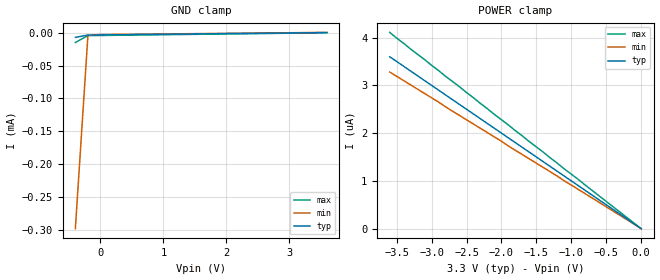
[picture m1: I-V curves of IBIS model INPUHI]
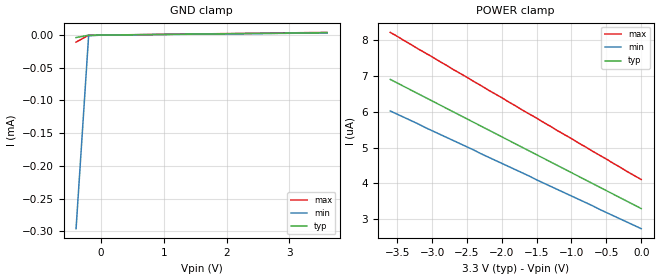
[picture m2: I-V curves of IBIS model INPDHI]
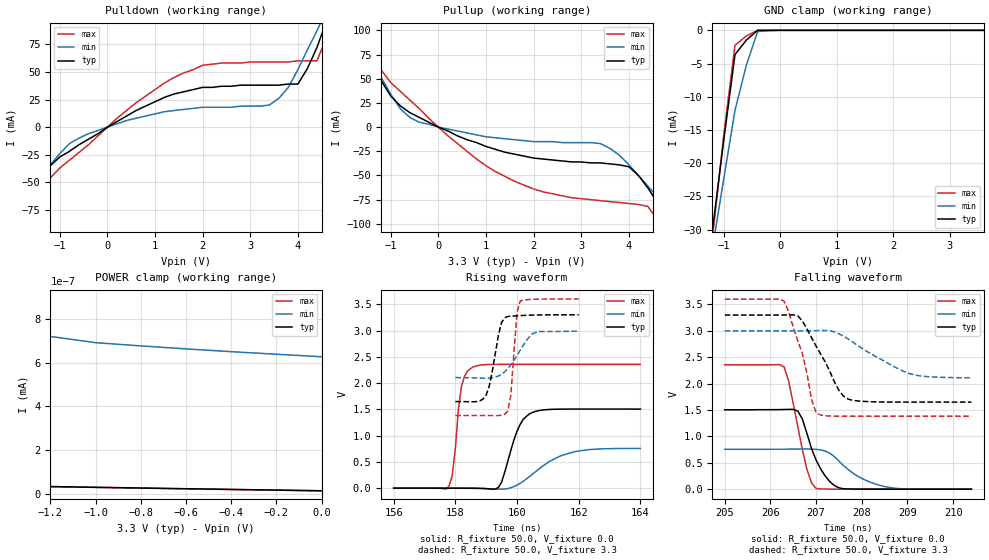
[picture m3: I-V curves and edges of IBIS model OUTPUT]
|   Texas Instruments Incorporated
|   Data Transmissions Products
|   IBIS Model for ISO723x4x
|   16DW SOIC Package
[IBIS Ver]   3.2
[Comment char]   |_char
[File name]   iso7240cf_3.ibs
[File Rev]   1.0
[Date]   10July08
[Source]   File originated at Texas Instruments Incorporated.
   Data Transmission Products Group.
[Notes]
[Disclaimer]
(C) Copyright Texas Instruments Incorporated 2002
   All rights reserved
  Texas Instruments Incorporated hereby grants the user of this IBIS
model a non-exclusive, nontransferable license to use this IBIS model
under the following terms.  Before using this IBIS model, the user
should read this license.  If the user does not accept these terms,
the IBIS model should be returned to Texas Instruments within 30 days.
  The user is granted this license only to use the IBIS model and
is not granted rights to sell, load, rent, lease or license the IBIS
model in whole or in part, or in modified form to anyone other than
user.  User may modify the IBIS model to suit its specific applications
but rights to derivative works and such modifications shall belong to
Texas Instruments.
  This IBIS model is provided on an "AS IS" basis and Texas Instruments
makes absolutely no warranty with respect to the information contained
herein.  TEXAS INSTRUMENTS DISCLAIMS AND CUSTOMER WAIVES ALL WARRANTIES,
EXPRESS OR IMPLIED, INCLUDING WARRANTIES OF MERCHANTABILITY OR FITNESS
FOR A PARTICULAR PURPOSE. The entire risk as to quality and performance
is with the Customer. ACCORDINGLY, IN NO EVENT SHALL THE COMPANY BE LIABLE
FOR ANY DAMAGES, WHETHER IN CONTRACT OR TORT,INCLUDING ANY LOST PROFITS
OR OTHER INCIDENTAL, CONSEQUENTIAL, EXEMPLARY, OR PUNITIVE DAMAGES ARISING
OUT OF THE USE OR APPLICATION OF THE IBIS model provided in this package.
Further, Texas Instruments reserves the right to discontinue or make changes
without notice to any product herein to improve reliability, function, or
design. Texas Instruments does not convey any license under patent rights
or any other intellectual property rights, including those of third parties.
Contact Texas Instruments at ATTN:DATA TRANSMISSIONS
[Copyright]   Copyright 2002, Texas Instruments, All Rights Reserved
[Component]   ISO7240DW
[Manufacturer]  Texas Instruments Incorporated
[Package]
|   typ   min   max
R_pkg   0.04817   0.03432   0.09530
L_pkg   2.4595nH   1.6904nH   4.7034nH
C_pkg   0.847pF   0.428pF   1.397pF
[Pin]   signal_name   model_name   R_pin   L_pin   C_pin
1   VCC1   POWER   0.03455  3.39778n  0.89677p
2   GND1   GND   0.03432  3.12613n  0.84706p
3   INA   INPUHI   0.04265  1.85523n  0.57831p
4   INB   INPUHI   0.03948  1.69049n  0.59300p
5   INC   INPUHI   0.03943  1.70546n  0.55709p
6   IND   INPUHI   0.04257  1.86953n  0.56379p
7   DISABLE   INPDHI   0.04783  1.99000n  0.60148p
8   GND1   GND   0.03740  4.70338n  1.39696p
9   GND2   GND   0.03763  4.61305n  1.39587p
10   CTRL   INPUHI   0.04703  2.01514n  0.58483p
11   OUTD   OUTPUT   0.07132  2.45946n  0.43321p
12   OUTC   OUTPUT   0.06147  2.13194n  0.42769p
13   OUTB   OUTPUT   0.07288  2.39260n  0.48001p
14   OUTA   OUTPUT   0.09530  3.03704n  0.47622p
15   GND2   GND   0.04817  4.23145n  0.93567p
16   VCC2   POWER   0.04790  4.51154n  0.99405p
| Models and submodels in the file (3): INPUHI (Input), INPDHI (Input), OUTPUT (3-state)
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|   Driver Enable
[Model]   INPUHI
Model_type   Input
|Signals   INA,INB,INC,IND,CTRL
Vinh = 2.0
Vinl = 0.8
|   typ   min   max
C_comp   1.3pF   1.1pF   1.5pF
|   typ   min   max
[Temperature Range]   27   -40   125
[Voltage range]   3.3V   3.0V   3.6V
[GND_clamp]
|   Voltage   I(typ)   I(min)   I(max)
-400mV    -7.04uA    -298uA     -14.8uA
-200mV    -3.5uA     -3.91uA    -4.34uA
0V        -3.3uA     -2.74uA    -4.11uA
3.6V      300nA      549nA      14.4pA
[Power_clamp]
| Note that the[POWER_clamp]voltage table is referenced to Vcc
| and is calculated using Vtable=Vcc - Vmeasured.
|   Voltage   I(typ)   I(min)   I(max)
-3.6V     3.6uA      3.28uA     4.11uA
-2.9V     2.9uA      2.65uA     3.31uA
-2.8V     2.8uA      2.55uA     3.19uA
0V        0A         0A         0A
|   Driver Input / Receiver Enable Model
[Model]   INPDHI
Model_type   Input
|Signals   DISABLE
Vinh = 2.0
Vinl = 0.8
|   typ   min   max
C_comp   1.3pF   1.1pF   1.5pF
|   typ   min   max
[Temperature Range]   27   -40   125
[Voltage range]   3.3V   3.0V   3.6V
[GND_clamp]
|   Voltage   I(typ)   I(min)   I(max)
-400mV    -3.79uA    -296uA     -10.8uA
-200mV    -202nA     -1.2uA     -230nA
0V        0A         0A         0A
3.6V      3.6uA      3.28uA     4.11uA
[Power_clamp]
| Note that the[POWER_clamp]voltage table is referenced to Vcc
| and is calculated using Vtable=Vcc - Vmeasured.
|   Voltage   I(typ)   I(min)   I(max)
-3.6V     6.9uA      6.02uA     8.21uA
-500mV    3.8uA      3.19uA     4.68uA
-200mV    3.5uA      2.92uA     4.33uA
0V        3.3uA      2.74uA     4.11uA
[Model]   OUTPUT
Model_type   3-state
| Signals   OUT
Vmeas = 2.2V   |Reference voltage for timing measurements
Cref = 15pF   |Timing specification test load capacitance value
Vref = 0   |Timing specification test load voltage; GND
| variable   typ   min   max
C_comp   2.1pF   1.7pF   2.5pF
|   typ   min   max
[Temperature Range]   25.0   -40   125
[Voltage range]   3.3V   3.0V   3.6V
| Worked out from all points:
|   slope of the pulldown table from 0 to 0.495 V, typ, clamps not added: 40 ohm
|   slope of the pullup table from 0 to 0.495 V, typ, clamps not added: 45.4 ohm
|   GND clamp passes 1 mA (typ) near -0.54 V on its own axis
|   POWER clamp passes 1 mA (typ) near -2.27 V on its own axis
|   rising waveform, R_fixture 50.0, V_fixture 0.0: 20-80 % time 494ps typ, 1.13ns min, 242ps max; typ from 0 V to 1.5 V
|   falling waveform, R_fixture 50.0, V_fixture 0.0: 20-80 % time 416ps typ, 716ps min, 336ps max; typ from 1.5 V to 0 V
|   rising waveform, R_fixture 50.0, V_fixture 3.3: 20-80 % time 308ps typ, 597ps min, 168ps max; typ from 1.65 V to 3.3 V
|   falling waveform, R_fixture 50.0, V_fixture 3.3: 20-80 % time 592ps typ, 1.04ns min, 405ps max; typ from 3.3 V to 1.65 V
[Pulldown]
|   Voltage  I(typ)   I(min)   I(max)
-3.6V     -213mA     -167mA     -286mA
-2.2V     -106mA     -89mA      -137mA
-1.8V     -76mA      -66mA      -95mA
-1.2V     -35mA      -34mA      -46mA
-600mV    -16mA      -10mA      -23mA
2V        36mA       18mA       56mA
3.4V      38mA       20mA       59mA
4V        39mA       52mA       60mA
4.4V      72mA       87mA       60mA
4.6V      96mA       106mA      81mA
4.8V      120mA      124mA      106mA
7.5V      465mA      379mA      575mA
[Pullup]
|   Voltage   I(typ)  I(min)  I(max)
| Note that the[Pullup]voltage table is referenced to Vcc
| and is calculated using Vtable=Vcc - Vmeasured.
-3.6V     345mA      272mA      457mA
-2V       144mA      123mA      182mA
-1.5V     83mA       78mA       100mA
-1.2V     48mA       51mA       59mA
-600mV    15mA       10mA       28mA
800mV     -16mA      -8mA       -33mA
2V        -32mA      -15mA      -64mA
3.4V      -37mA      -17mA      -76mA
4V        -41mA      -39mA      -79mA
4.4V      -63mA      -61mA      -82mA
5V        -108mA     -95mA      -134mA
7.2V      -281mA     -221mA     -373mA
[GND_clamp]
|   Voltage   I(typ)   I(min)   I(max)
| Outputs in High Impedance (off)
-3.6V     -213mA     -167.2mA   -285.4mA
-1.2V     -30.16mA   -32.94mA   -31.43mA
-1.1V     -23.41mA   -27.68mA   -23.65mA
-1V       -16.66mA   -22.42mA   -15.87mA
-800mV    -3.66mA    -12.05mA   -2.249mA
-600mV    -1.479mA   -5.279mA   -861.1uA
-400mV    -1.657uA   -187.7uA   -4.797uA
0V        -40.79pA   -10.95nA   -39.6pA
3.6V      17.57pA    663pA      12.68pA
[POWER_clamp]
|   Voltage  I(typ)   I(min)   I(max)
| Note that the [POWER_clamp] voltage table is referenced to Vcc
| and is calculated using Vtable = Vcc - Vmeasured.
| Outputs in Tri-state.
-3.6V     130.9mA    132.2mA    129.3mA
-2.2V     594.7uA    10.13mA    942.3pA
-2.1V     8.158nA    6.126mA    495.1pA
-2V       5.434nA    2.119mA    47.98pA
-1.8V     1.376nA    388.9uA    43.35pA
-1.7V     41.24pA    194.6uA    41.32pA
-1.5V     37.53pA    132.3nA    37.35pA
-1.4V     35.76pA    755.1pA    35.42pA
-1.2V     32.25pA    720.1pA    31.79pA
-1V       28.85pA    691.4pA    28.37pA
-400mV    19.15pA    650.1pA    18.72pA
0V        12.94pA    627pA      12.68pA
[Ramp]
|   typ   min   max
dV/dt_r   0.903V/0.494ns   0.454V/1.13ns   1.414V/0.242ns
dV/dt_f   0.903V/0.416ns   0.453V/0.717ns  1.414V/0.336ns
R_load = 50
[Rising Waveform]
R_fixture = 50.0
V_fixture = 0.0
C_fixture = 0p
L_fixture = 0n
|   V(typ)   V(min)   V(max)
156ns     489.7pV    12.09nV    431.9pV
157.8ns   17.01uV    282.3uV    42.76mV
157.9ns   27.86uV    217.4uV    238.3mV
158.2ns   89.93uV    -788.4uV   1.94V
158.6ns   -99.63uV   -4.419mV   2.312V
159.4ns   15.91mV    -17.3mV    2.357V
160ns     1.083V     58.82mV    2.357V
160.5ns   1.441V     266mV      2.357V
161.9ns   1.506V     698.7mV    2.357V
164ns     1.505V     756mV      2.357V
[Falling Waveform]
R_fixture = 50.0
V_fixture = 0.0
C_fixture = 0p
L_fixture = 0n
|   V(typ)   V(min)   V(max)
205ns     1.505V     755.2mV    2.357V
206.3ns   1.51V      757.4mV    2.318V
206.4ns   1.512V     758.3mV    2.047V
206.6ns   1.481V     760.6mV    1.187V
206.8ns   1.057V     762mV      375.6mV
207ns     553.1mV    755.1mV    12.03mV
207.3ns   143.1mV    683mV      796.9uV
207.6ns   7.515mV    447.7mV    36.71uV
208.5ns   197.3uV    48.97mV    -2.819uV
210.4ns   -4.04uV    324.3uV    303.2nV
[Rising Waveform]
R_fixture = 50.0
V_fixture = 3.3
V_fixture_min = 3.0
V_fixture_max = 3.6
C_fixture = 0p
L_fixture = 0n
|   V(typ)   V(min)  V(max)
158ns     1.649V     2.106V     1.383V
159ns     1.774V     2.093V     1.382V
159.1ns   1.943V     2.094V     1.382V
159.5ns   3.156V     2.171V     1.389V
159.7ns   3.268V     2.277V     1.468V
159.8ns   3.274V     2.348V     1.768V
160ns     3.282V     2.527V     3.341V
160.1ns   3.285V     2.625V     3.559V
160.6ns   3.296V     2.964V     3.597V
162ns     3.3V       2.989V     3.6V
[Falling Waveform]
R_fixture = 50.0
V_fixture = 3.3
V_fixture_min = 3.0
V_fixture_max = 3.6
C_fixture = 0p
L_fixture = 0n
|   V(typ)   V(min)  V(max)
205ns     3.3V       3V         3.6V
206.3ns   3.3V       3V         3.563V
206.6ns   3.286V     3V         2.812V
206.7ns   3.187V     3V         2.569V
206.9ns   2.874V     3.002V     1.705V
207.1ns   2.561V     3.006V     1.404V
207.5ns   1.872V     2.947V     1.383V
207.7ns   1.707V     2.846V     1.383V
209ns     1.65V      2.201V     1.383V
210.4ns   1.65V      2.11V      1.383V
